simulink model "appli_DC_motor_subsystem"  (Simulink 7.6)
settings: Solver=ode15s  StartTime=0.0  StopTime=N  RelTol=1e-3
PreLoadFcn:
  | clc, close all,, delete *.mat
InitFcn:
  | N=1e-5
StopFcn:
  | clc, close all, delete *.mat
  | load Signaux_DC_motor.mat
  | 
  | subplot 121
  | plot(x(1,:),x(2,:))
  | 
  | 
  | plot(x(1,:), x(3,:))
  | hold on
  | plot(x(1,:), x(2,:))
  | grid
  | 
  | subplot 122
  | plot(x(1,:), x(4,:))
libraries: fl_lib x12, nesl_utility x5, powerlib_extras x1

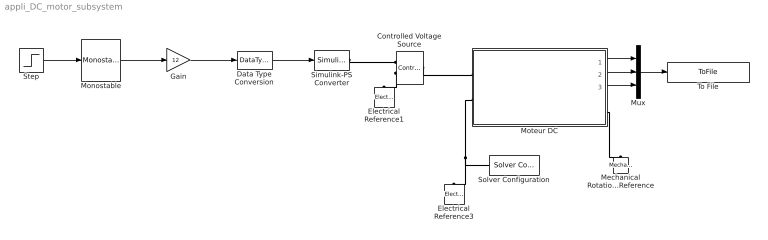
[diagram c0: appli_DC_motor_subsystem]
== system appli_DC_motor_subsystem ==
  Controlled Voltage Source : fl_lib/Electrical/Electrical Sources/Controlled Voltage Source  DialogController=NetworkEngine.DynNeDlgSource  SystemSampleTime=-1  i_Log=off  v_Log=off  LocalVarNames=|current|voltage|power  LocalVarDescs=|Current (A)|Voltage (V)|Power (W)  LocalVarLogging=[0 0 0]
  Data Type Conversion : DataTypeConversion  OutDataTypeStr=double
  Electrical Reference1 : fl_lib/Electrical/Electrical Elements/Electrical Reference  DialogController=NetworkEngine.DynNeDlgSource  SystemSampleTime=-1  i_Log=off  LocalVarNames=|i  LocalVarDescs=|i  LocalVarLogging=[]
  Electrical Reference3 : fl_lib/Electrical/Electrical Elements/Electrical Reference  DialogController=NetworkEngine.DynNeDlgSource  SystemSampleTime=-1  i_Log=off  LocalVarNames=|i  LocalVarDescs=|i  LocalVarLogging=[]
  Gain : Gain  Gain=12
  Mechanical Rotational Reference : fl_lib/Mechanical/Rotational Elements/Mechanical Rotational Reference  DialogController=NetworkEngine.DynNeDlgSource  SystemSampleTime=-1  t_Log=off  LocalVarNames=|t  LocalVarDescs=|t  LocalVarLogging=[]
  Monostable : powerlib_extras/Control  Blocks/Monostable  DialogController=POWERSYS.PowerSysDialog  SystemSampleTime=-1  EdgeDetect=Rising  t_mono=N  ic=0
  Moteur DC : Subsystem
  Mux : Mux  Inputs=3
  Simulink-PS Converter : nesl_utility/Simulink-PS Converter  DialogController=NetworkEngine.DynNeUtilDlgSource  SystemSampleTime=-1  PhysicalDomain=network_engine_domain  LeftPortType=input  RightPortType=output  SubClassName=ps_input  Unit=1  AffineConversion=off  InputFilterTimeConstant=.001  UdotUserProvided=0
  Solver Configuration : nesl_utility/Solver Configuration  DialogController=NetworkEngine.DynNeUtilDlgSource  SystemSampleTime=-1  PhysicalDomain=network_engine_domain  LeftPortType=input  RightPortType=generic  SubClassName=solver  Accelerate=off  Profile=off  ResidualTolerance=1e-9  MaxNonlinIter=12  MaxModeIter=2  DoFixedCost=off  UseLocalSampling=off  DoDC=off  LinearAlgebra=Sparse  LocalSolverSampleTime=.001  LocalSolverChoice=NE_BACKWARD_EULER_ADVANCER  UseLocalSolver=off
  Step : Step  SampleTime=0
  To File : ToFile  Filename=Signaux_DC_motor  MatrixName=x
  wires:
  Moteur DC/1(I_nduit) -> Mux/1
  Moteur DC/2(vitesse) -> Mux/2
  Moteur DC/3(Angle) -> Mux/3
  Mux/1 -> To File/1
  Monostable/1 -> Gain/1
  Step/1 -> Monostable/1
  Data Type Conversion/1 -> Simulink-PS Converter/1
  Gain/1 -> Data Type Conversion/1
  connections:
  Moteur DC/RConn2 -- Mechanical Rotational Reference/LConn1
  Moteur DC/LConn2 -- Electrical Reference3/LConn1 -- Solver Configuration/RConn1
  Simulink-PS Converter/RConn1 -- Controlled Voltage Source/RConn1
  Controlled Voltage Source/LConn1 -- Moteur DC/LConn1
  Controlled Voltage Source/RConn2 -- Electrical Reference1/LConn1

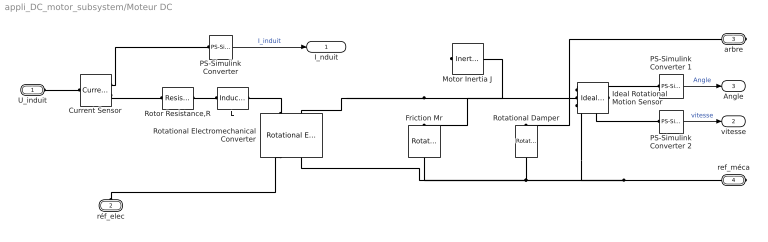
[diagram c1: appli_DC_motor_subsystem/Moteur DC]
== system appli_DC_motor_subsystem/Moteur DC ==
  Current Sensor : fl_lib/Electrical/Electrical Sensors/Current Sensor  DialogController=NetworkEngine.DynNeDlgSource  SystemSampleTime=-1  i1_Log=off  v1_Log=off  LocalVarNames=|i1|v1  LocalVarDescs=|i1|v1  LocalVarLogging=[0 0]
  Friction Mr : fl_lib/Mechanical/Rotational Elements/Rotational Friction  DialogController=NetworkEngine.DynNeDlgSource  SystemSampleTime=-1  brkwy_trq=0.02e-3 N*m  Col_trq=0.02e-3 N*m  visc_coef=0 N*m/(rad/s)  trans_coef=10 s/rad  vel_thr=0.1 rad/s  t_Log=off  w_Log=off  LocalVarNames=|friction_torque|rel_velocity|power  LocalVarDescs=|Friction torque (N*m)|Relative velocity (rad/s)|Power (W)  LocalVarLogging=[0 0 0]
  Ideal Rotational Motion Sensor : fl_lib/Mechanical/Mechanical Sensors/Ideal Rotational Motion Sensor  DialogController=NetworkEngine.DynNeDlgSource  SystemSampleTime=-1  offset=0 rad  w_Log=off  t_Log=off  phi_Log=off  LocalVarNames=|w|t|phi  LocalVarDescs=|w|t|phi  LocalVarLogging=[]
  L : fl_lib/Electrical/Electrical Elements/Inductor  DialogController=NetworkEngine.DynNeDlgSource  SystemSampleTime=-1  l=12e-6 H  i0=0 A  r=0 Ohm  g=1e-09 1/Ohm  i_Log=off  v_Log=off  i_L_Log=off  LocalVarNames=|current|voltage|power  LocalVarDescs=|Inductor current (A) |Voltage across inductor (V)|Power (W)  LocalVarLogging=[0 0 0]
  Motor Inertia J : fl_lib/Mechanical/Rotational Elements/Inertia  DialogController=NetworkEngine.DynNeDlgSource  SystemSampleTime=-1  inertia=0.01 g*cm^2  initial_velocity=0 rad/s  t_Log=off  LocalVarNames=|torque|velocity  LocalVarDescs=|Inertia torque (N*m)|Inertia absolute velocity (rad/s)  LocalVarLogging=[0 0]
  PS-Simulink Converter : nesl_utility/PS-Simulink Converter  DialogController=NetworkEngine.DynNeUtilDlgSource  SystemSampleTime=-1  PhysicalDomain=network_engine_domain  LeftPortType=input  RightPortType=output  SubClassName=ps_output  Unit=1  AffineConversion=off
  PS-Simulink Converter 1 : nesl_utility/PS-Simulink Converter  DialogController=NetworkEngine.DynNeUtilDlgSource  SystemSampleTime=-1  PhysicalDomain=network_engine_domain  LeftPortType=input  RightPortType=output  SubClassName=ps_output  Unit=rad  AffineConversion=off
  PS-Simulink Converter 2 : nesl_utility/PS-Simulink Converter  DialogController=NetworkEngine.DynNeUtilDlgSource  SystemSampleTime=-1  PhysicalDomain=network_engine_domain  LeftPortType=input  RightPortType=output  SubClassName=ps_output  Unit=rpm  AffineConversion=off
  Rotational Electromechanical Converter : fl_lib/Electrical/Electrical Elements/Rotational Electromechanical Converter  DialogController=NetworkEngine.DynNeDlgSource  SystemSampleTime=-1  K=0.072e-3*60/(2*pi) V/(rad/s)  i_Log=off  v_Log=off  t_Log=off  w_Log=off  LocalVarNames=|current|voltage|power|torque|speed  LocalVarDescs=|Current (A)|Voltage (V)|Power (W)|Torque (Nm)|Angular speed (rad/s)  LocalVarLogging=[0 0 0 0 0]
  Rotational Damper : fl_lib/Mechanical/Rotational Elements/Rotational Damper  DialogController=NetworkEngine.DynNeDlgSource  SystemSampleTime=-1  D=0.001 N*m/(rad/s)  t_Log=off  w_Log=off  LocalVarNames=|t|w  LocalVarDescs=|t|w  LocalVarLogging=[0 0]
  Rotor Resistance,R : fl_lib/Electrical/Electrical Elements/Resistor  Tag=Factory Generic  DialogController=NetworkEngine.DynNeDlgSource  SystemSampleTime=-1  R=3.9 Ohm  i_Log=off  v_Log=off  LocalVarNames=|current|voltage|power  LocalVarDescs=|Resistor current (A)|Voltage across resistor (V)|Power (W)  LocalVarLogging=[0 0 0]
  U_induit : PMIOPort  Port=1  Side=Left
  réf_elec : PMIOPort  Port=2  Side=Left
  arbre : PMIOPort  Port=3  Side=Right
  ref_méca : PMIOPort  Port=4  Side=Right
  I_nduit : Outport
  vitesse : Outport  Port=2
  Angle : Outport  Port=3
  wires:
  PS-Simulink Converter 2/1 -> vitesse/1  "vitesse"
  PS-Simulink Converter 1/1 -> Angle/1  "Angle"
  PS-Simulink Converter/1 -> I_nduit/1  "I_induit"
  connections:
  réf_elec/RConn1 -- Rotational Electromechanical Converter/RConn1
  U_induit/RConn1 -- Current Sensor/LConn1
  Rotational Electromechanical Converter/LConn1 -- L/RConn1
  L/LConn1 -- Rotor Resistance,R/RConn1
  Ideal Rotational Motion Sensor/RConn3 -- PS-Simulink Converter 1/LConn1
  Ideal Rotational Motion Sensor/RConn2 -- PS-Simulink Converter 2/LConn1
  Ideal Rotational Motion Sensor/RConn1 -- Rotational Damper/RConn1 -- Rotational Electromechanical Converter/RConn2 -- Friction Mr/RConn1 -- ref_méca/RConn1
  Ideal Rotational Motion Sensor/LConn1 -- Rotational Damper/LConn1 -- Friction Mr/LConn1 -- Rotational Electromechanical Converter/LConn2 -- Motor Inertia J/LConn1 -- arbre/RConn1
  Current Sensor/RConn2 -- Rotor Resistance,R/LConn1
  Current Sensor/RConn1 -- PS-Simulink Converter/LConn1
